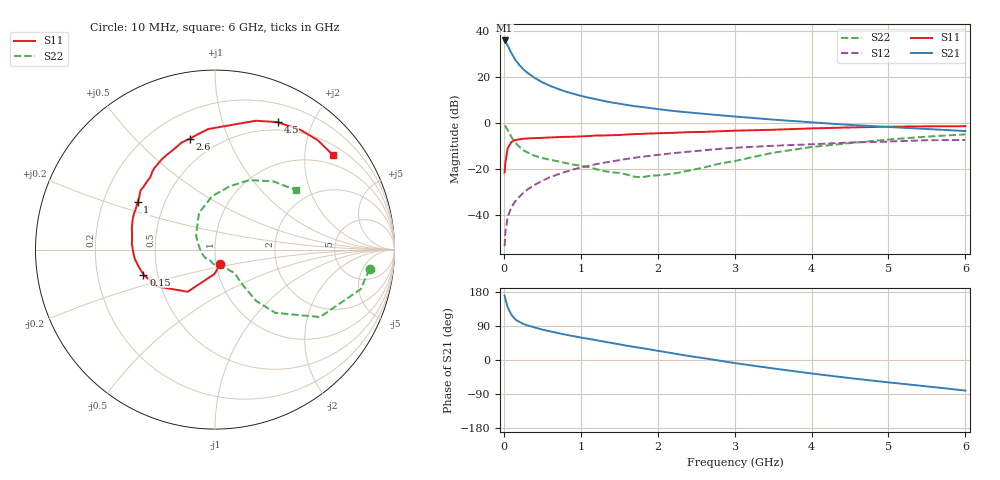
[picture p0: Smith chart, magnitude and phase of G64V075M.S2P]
! SIEMENS Small Signal Semiconductors
! BFG193
! Si NPN RF Bipolar Junction Transistor in SOT223
! VCE = 4 V  IC = 75 mA
! Common Emitter S-Parameters:  August  1996
# GHz  S  MA  R  50
!  f  S11  S21  S12  S22
! GHz  MAG  ANG  MAG  ANG  MAG  ANG  MAG  ANG
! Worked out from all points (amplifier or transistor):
!   36 points, 10 MHz to 6 GHz, reference 50 ohm
!   highest |S21| = 35.7 dB at 10 MHz (marker M1)
!   |S21| within 3 dB of that: start of sweep to 62.09 MHz
!   unconditionally stable (mu >= 1): 311.7 MHz to 2.371 GHz
!   at 250 MHz: K = 0.98, MSG = 26.9 dB, |S12| = -30.5 dB
!   at 1.4 GHz: K = 1.06, MAG = 11.3 dB, |S12| = -16.8 dB
!   at 6 GHz: K = 0.91, MSG = 1.9 dB, |S12| = -7.5 dB
!   S11 on the Smith chart (normalised r, x): 10 MHz: 1.05, -0.17; 150 MHz: 0.42, -0.14; 1 GHz: 0.35, +0.25; 2.6 GHz: 0.36, +0.73; 4.5 GHz: 0.40, +1.53; 6 GHz: 0.74, +2.67
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0.01  0.0839 -69.1  61 170.0  0.0021 83.0  0.8678 -7.2
0.02  0.136 -91.3  58.19 161.2  0.0042 75.9  0.8411 -15.2
0.05  0.2801 -123.0  47.46 138.8  0.0091 69.5  0.6956 -32.7
0.1  0.3845 -147.8  32.12 118.9  0.0149 68.8  0.4863 -46.4
0.15  0.4224 -160.8  23.15 107.1  0.0199 68.7  0.3665 -51.3
0.2  0.4355 -167.3  18.08 100.7  0.0247 70.2  0.3021 -51.6
0.25  0.4499 -173.4  14.67 95.6  0.0297 70.8  0.2555 -51.8
0.3  0.4557 -177.8  12.38 91.7  0.0349 71.4  0.2306 -51.8
0.4  0.4642 176.0  9.408 85.9  0.0448 71.3  0.1925 -50.8
0.5  0.47 169.4  7.545 80.2  0.0552 70.6  0.1707 -50.4
0.6  0.4796 165.1  6.331 75.7  0.0658 68.9  0.1583 -51.7
0.8  0.4938 156.3  4.766 67.1  0.086 65.5  0.1335 -56.4
1  0.5052 148.6  3.845 59.4  0.1064 61.8  0.1172 -62.5
1.1  0.5137 145.3  3.504 55.9  0.1158 60.2  0.1091 -68.5
1.3  0.5303 138.7  2.977 48.5  0.1358 56.1  0.0895 -78.2
1.6  0.5562 129.0  2.427 37.6  0.1645 49.0  0.0751 -102.9
2.2  0.604 112.4  1.806 17.6  0.2189 35.4  0.0782 -167.9
2.6  0.6339 102.8  1.565 4.8  0.2527 26.5  0.1068 154.9
3.5  0.7047 81.4  1.17 -22.2  0.3166 3.7  0.2236 113.4
4.5  0.7913 63.8  0.897 -47.8  0.3724 -16.5  0.3622 76.9
5.5  0.8362 46.8  0.732 -69.7  0.4174 -40.2  0.4999 49.5
6  0.8422 38.7  0.66 -80.6  0.4222 -53.7  0.5597 36.3
